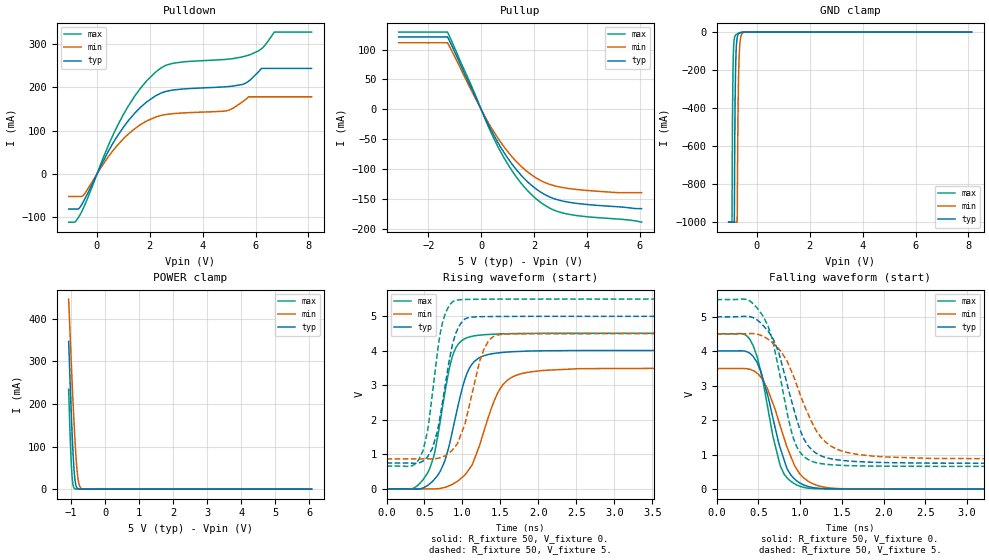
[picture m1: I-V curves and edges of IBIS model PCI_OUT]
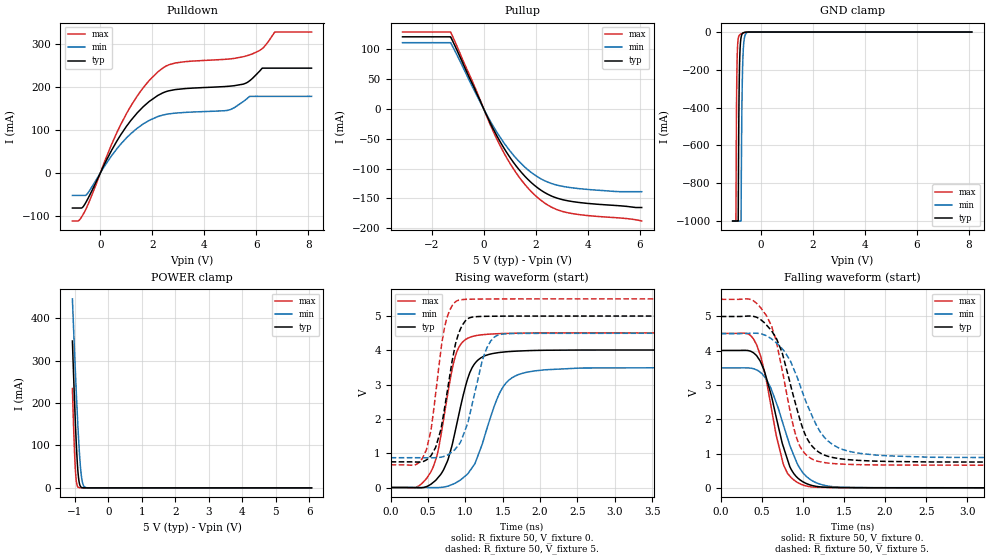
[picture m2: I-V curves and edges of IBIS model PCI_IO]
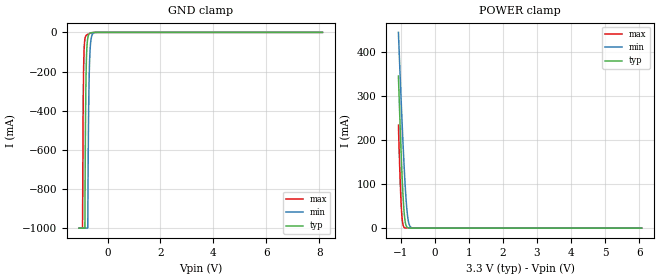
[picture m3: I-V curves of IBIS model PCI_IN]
|   IBIS Model for tsi381
[IBIS Ver]   3.2
[Disclaimer] THIS IBIS MODEL HAS BEEN CREATED BY THE SIGNAL
   INTEGRITY SOFTWARE SPICE-TO-IBIS PROCESS.
   THESE IBIS MODELS ARE PROVIDED "AS IS" WITH NO
   WARRANTY WHATSOEVER AND SIGNAL INTEGRITY SOFTWARE
   SPECIFICALLY DISCLAIMS ANY IMPLIED WARRANTIES OF
   MERCHANTABILITY, FITNESS FOR A PARTICULAR PURPOSE,
   OR AGAINST INFRINGEMENT.
[File Name]   tsi381_pbga_5vpci.ibs
[File Rev]   1.1
[Date]   07/27/2009
[Notes]
   Revision History
   Rev 1.0
   - 2/27/09 Inital Release. IBIS model generated from
   SPICE model extraction. AEP
   Rev 1.1
   - updated it IDT formating. IGT
[Component] tsi381
[Manufacturer] IDT
|   typ   min   max
[Package]
R_pkg   354m   244m   481m
L_pkg   4.50nH   2.81nH   7.01nH
C_pkg   0.86pF   0.64pF   1.33pF
[Pin]  signal_name   model_name   R_pin   L_pin   C_pin
C9   GPIO[0]   NC   299.8m   3.7nh   0.83pf
A10   GPIO[1]   NC   274.4m   3.5nh   0.76pf
B10   GPIO[2]   NC   247.9m   3.3nh   0.64pf
A11   GPIO[3]   NC   287.0m   3.6nh   0.79pf
M2   JTAG_TCK   JTAG_IN   366.2m   4.4nh   0.83pf
L3   JTAG_TDI   JTAG_IN   382.4m   4.9nh   0.94pf
L1   JTAG_TDO   JTAG_OUT   371.7m   4.5nh   0.76pf
M12   JTAG_TMS   JTAG_IN   393.2m   4.5nh   0.85pf
L10   JTAG_TRSTn   JTAG_IN   410.4m   5.3nh   0.96pf
D3   PCI_AD[0]   PCI_IO   398.2m   5.4nh   0.99pf
C1   PCI_AD[1]   PCI_IO   344.1m   4.1nh   0.77pf
F4   PCI_AD[10]   PCI_IO   402.7m   5.8nh   1.06pf
G1   PCI_AD[11]   PCI_IO   310.8m   3.7nh   0.64pf
G2   PCI_AD[12]   PCI_IO   330.2m   4.0nh   0.77pf
G3   PCI_AD[13]   PCI_IO   375.2m   4.9nh   0.90pf
H1   PCI_AD[14]   PCI_IO   311.3m   3.8nh   0.65pf
H2   PCI_AD[15]   PCI_IO   355.7m   4.5nh   0.82pf
J5   PCI_AD[16]   PCI_IO   481.4m   6.8nh   1.29pf
L6   PCI_AD[17]   PCI_IO   343.6m   4.4nh   0.79pf
M6   PCI_AD[18]   PCI_IO   304.3m   3.8nh   0.66pf
K6   PCI_AD[19]   PCI_IO   371.5m   5.1nh   0.92pf
D1   PCI_AD[2]   PCI_IO   330.9m   3.9nh   0.72pf
J6   PCI_AD[20]   PCI_IO   386.3m   5.7nh   1.04pf
M7   PCI_AD[21]   PCI_IO   301.3m   3.7nh   0.65pf
L7   PCI_AD[22]   PCI_IO   326.6m   4.1nh   0.77pf
K7   PCI_AD[23]   PCI_IO   373.6m   4.9nh   0.92pf
L8   PCI_AD[24]   PCI_IO   357.1m   4.4nh   0.81pf
K8   PCI_AD[25]   PCI_IO   437.6m   5.8nh   1.12pf
M9   PCI_AD[26]   PCI_IO   323.3m   3.9nh   0.69pf
L9   PCI_AD[27]   PCI_IO   357.9m   4.5nh   0.84pf
K12   PCI_AD[28]   PCI_IO   346.8m   4.1nh   0.79pf
J11   PCI_AD[29]   PCI_IO   377.8m   4.7nh   0.93pf
D2   PCI_AD[3]   PCI_IO   353.3m   4.5nh   0.85pf
J12   PCI_AD[30]   PCI_IO   324.4m   4.0nh   0.74pf
J10   PCI_AD[31]   PCI_IO   436.5m   5.9nh   1.16pf
E1   PCI_AD[4]   PCI_IO   309.0m   3.7nh   0.67pf
E2   PCI_AD[5]   PCI_IO   352.5m   4.6nh   0.82pf
E3   PCI_AD[6]   PCI_IO   368.0m   5.0nh   0.94pf
E4   PCI_AD[7]   PCI_IO   480.4m   7.0nh   1.32pf
F2   PCI_AD[8]   PCI_IO   343.3m   4.2nh   0.79pf
F3   PCI_AD[9]   PCI_IO   363.1m   4.8nh   0.91pf
F1   PCI_CBEn[0]   PCI_IO   303.6m   3.7nh   0.65pf
H3   PCI_CBEn[1]   PCI_IO   392.2m   5.0nh   0.94pf
K5   PCI_CBEn[2]   PCI_IO   406.7m   5.4nh   1.06pf
M8   PCI_CBEn[3]   PCI_IO   309.0m   3.8nh   0.66pf
D12   PCI_CLK   PCI_IN   328.4m   3.9nh   0.67pf
H10   PCI_CLKO[0]   PCI_OUT   407.4m   5.6nh   1.09pf
C2   PCI_CLKO[1]   PCI_OUT   408.8m   5.2nh   0.95pf
K4   PCI_DEVSELn   PCI_IO   467.5m   6.4nh   1.28pf
M5   PCI_FRAMEn   PCI_IO   317.2m   3.8nh   0.68pf
G10   PCI_GNTn[0]   PCI_IO   377.6m   4.9nh   1.01pf
G9   PCI_GNTn[1]   PCI_OUT   404.4m   5.5nh   1.09pf
F11   PCI_GNTn[2]   PCI_OUT   346.6m   4.4nh   0.82pf
E11   PCI_GNTn[3]   PCI_OUT   340.9m   4.1nh   0.79pf
E12   PCI_INTAn   PCI_IN   321.7m   4.0nh   0.66pf
E9   PCI_INTBn   PCI_IN   395.4m   5.5nh   1.06pf
D11   PCI_INTCn   PCI_IN   380.1m   4.7nh   0.82pf
E10   PCI_INTDn   PCI_IN   390.8m   5.0nh   0.93pf
L5   PCI_IRDYn   PCI_IO   351.2m   4.5nh   0.87pf
M3   PCI_LOCKn   PCI_OUT   333.8m   4.2nh   0.69pf
D10   PCI_M66EN   PCI_IN   420.4m   5.6nh   0.97pf
J1   PCI_PAR   PCI_IO   328.0m   4.0nh   0.66pf
J3   PCI_PERRn   PCI_IO   436.6m   5.7nh   1.06pf
H12   PCI_PMEn   PCI_IN   326.8m   3.9nh   0.74pf
G11   PCI_REQn[0]   PCI_IO   348.8m   4.3nh   0.85pf
H9   PCI_REQn[1]   PCI_IN   420.8m   6.1nh   1.09pf
G12   PCI_REQn[2]   PCI_IN   305.3m   3.7nh   0.68pf
H11   PCI_REQn[3]   PCI_IN   335.4m   4.3nh   0.81pf
F10   PCI_RSTn   PCI_OUT   366.0m   4.9nh   0.90pf
J2   PCI_SERRn   PCI_IO   376.6m   4.8nh   0.83pf
L4   PCI_STOPn   PCI_IO   385.4m   4.9nh   0.95pf
M4   PCI_TRDYn   PCI_IO   326.3m   3.9nh   0.74pf
B12   PCIE_PERSTn   NC   347.3m   4.3nh   0.66pf
B6   PCIE_REFCLK_n   NC   339.4m   4.2nh   1.02pf
A6   PCIE_REFCLK_p   NC   341.4m   4.1nh   1.01pf
B7   PCIE_RXD_n   NC   253.1m   3.1nh   0.75pf
A8   PCIE_RXD_p   NC   266.3m   3.4nh   0.79pf
A4   PCIE_TXD_n   NC   249.7m   3.3nh   0.69pf
B5   PCIE_TXD_p   NC   244.8m   3.0nh   0.69pf
K11   PWRUP_EN_ARB   GEN33_IN   407.8m   5.1nh   1.04pf
M1   PWRUP_PLL_BYPASS   GEN33_IN   410.2m   4.8nh   0.93pf
B2   SR_CLK   NC   418.6m   5.1nh   0.96pf
C4   SR_CSn   NC   412.7m   5.5nh   1.33pf
A2   SR_DIN   NC   308.5m   3.8nh   0.87pf
A1   SR_DOUT   NC   366.1m   4.5nh   0.78pf
C8   TEST_BCE   NC   313.4m   4.3nh   0.96pf
B1   TEST_BIDR_CTL   NC   371.0m   4.4nh   0.80pf
A3   TEST_ON   NC   332.2m   4.3nh   0.93pf
M11   TEST_SPARE[0]   NC   371.4m   4.4nh   0.79pf
D8   TEST_SPARE[1]   NC   252.7m   2.8nh   0.70pf
K1   TEST_SPARE[2]   NC   349.1m   4.3nh   0.71pf
C10   VDD   POWER
D4   VDD   POWER
F6   VDD   POWER
F8   VDD   POWER
G6   VDD   POWER
G7   VDD   POWER
J9   VDD   POWER
K3   VDD   POWER
B3   VDD_PCI   POWER
B11   VDD_PCI   POWER
F9   VDD_PCI   POWER
G4   VDD_PCI   POWER
H5   VDD_PCI   POWER
H8   VDD_PCI   POWER
J7   VDD_PCI   POWER
L2   VDD_PCI   POWER
M10   VDD_PCI   POWER
A5   VDD_PCIE   POWER
A7   VDD_PCIE   POWER
D5   VDD_PCIE   POWER
E5   VDDA_PCIE   POWER
E7   VDDA_PLL   POWER
F5   VIO_PCI   POWER
G8   VIO_PCI   POWER
H6   VIO_PCI   POWER
B8   VSS   GND
B4   VSS   GND
C6   VSS   GND
C5   VSS   GND
D9   VSS   GND
D7   VSS   GND
D6   VSS   GND
E6   VSS   GND
F7   VSS   GND
G5   VSS   GND
H7   VSS   GND
H4   VSS   GND
A12   VSS_IO   GND
C11   VSS_IO   GND
C3   VSS_IO   GND
F12   VSS_IO   GND
J8   VSS_IO   GND
J4   VSS_IO   GND
K10   VSS_IO   GND
K2   VSS_IO   GND
C7   VSSA_PLL   GND
| Models and submodels in the file (6): PCI_OUT (Output), PCI_IO (I/O), PCI_IN (Input), JTAG_IN (Input), JTAG_OUT (Output), GEN33_IN (Input)
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[Model]   PCI_OUT
Model_type  Output
C_comp 4.536p 4.202p 4.874p
Polarity   Non-Inverting
Enable   Active-High
Vmeas =   1.32V
Cref =   10pF
Rref =   50
Vref=   0.0V
[Temperature Range]   27.0   125.0   -40.0
[Voltage Range] 5. 4.5 5.5
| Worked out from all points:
|   slope of the pulldown table from 0 to 0.75 V, typ, clamps not added: 8.81 ohm
|   slope of the pullup table from 0 to 0.75 V, typ, clamps not added: 11.8 ohm
|   GND clamp passes 1 mA (typ) near -0.58 V on its own axis
|   POWER clamp passes 1 mA (typ) near -0.80 V on its own axis
|   rising waveform, R_fixture 50, V_fixture 0.: 20-80 % time 271ps typ, 341ps min, 223ps max; typ from 0 V to 4.01 V
|   rising waveform, R_fixture 50, V_fixture 5.: 20-80 % time 204ps typ, 254ps min, 174ps max; typ from 0.748 V to 5 V
|   falling waveform, R_fixture 50, V_fixture 0.: 20-80 % time 260ps typ, 305ps min, 229ps max; typ from 4.01 V to 0 V
|   falling waveform, R_fixture 50, V_fixture 5.: 20-80 % time 307ps typ, 393ps min, 259ps max; typ from 5 V to 0.748 V
[Pulldown]
-1.072V   -80.93mA   -51.78mA   -111mA
-830.1mV  -80.93mA   -51.78mA   -110.2mA
-625.6mV  -75.05mA   -51.78mA   -92.1mA
425mV     51.67mA    39.35mA    65.16mA
1.011V    108.6mA    81.72mA    138.1mA
2.21V     179.7mA    130.8mA    234.1mA
2.879V    193.3mA    138.9mA    254.9mA
4.887V    200.8mA    145.2mA    263.9mA
5.761V    214.7mA    177.7mA    274.1mA
6.226V    243mA      177.7mA    288.2mA
6.71V     243mA      177.7mA    326.7mA
8.123V    243mA      177.7mA    326.7mA
[Pullup]
-3.123V   121mA      111.2mA    129.1mA
-1.273V   121mA      111.2mA    129.1mA
-408.1mV  39.21mA    34.71mA    43.33mA
103.2mV   -9.96mA    -8.61mA    -11.21mA
754mV     -64.09mA   -55.48mA   -71.94mA
1.433V    -105.7mA   -91.4mA    -118.6mA
1.786V    -121.9mA   -105.2mA   -136.8mA
2.186V    -135.9mA   -116.9mA   -152.8mA
2.725V    -148.2mA   -126.7mA   -167.3mA
3.264V    -154.4mA   -131.5mA   -174.5mA
4.984V    -161.7mA   -138.3mA   -182.2mA
6.072V    -165.4mA   -138.8mA   -188mA
[GND Clamp]
-1.072V   -1A        -1A        -1A
-946.2mV  -1A        -1A        -1A
-927.6mV  -1A        -1A        -477.7mA
-913.6mV  -1A        -1A        -259.6mA
-857.8mV  -1A        -1A        -35.04mA
-829.9mV  -387.1mA   -1A        -20.17mA
-792.7mV  -109.1mA   -1A        -13.52mA
-750.8mV  -31.16mA   -1A        -10.02mA
-718.2mV  -13.49mA   -425.6mA   -7.927mA
-681mV    -5.936mA   -150.7mA   -5.835mA
-541.4mV  -487.9uA   -4.567mA   -875.4uA
8.123V    0A         0A         0A
[Power Clamp]
-1.072V   346.3mA    445.7mA    234.2mA
-1.025V   239mA      352.7mA    117.5mA
-985.9mV  158.9mA    279.6mA    47.19mA
-953.7mV  100.9mA    221.8mA    15.32mA
-930mV    65.56mA    181.6mA    5.554mA
-906.4mV  38.32mA    144mA      1.868mA
-865.6mV  11.54mA    86.96mA    261.8uA
-839.8mV  4.741mA    57.78mA    114.1uA
-809.7mV  1.564mA    32.24mA    114.1uA
-764.6mV  288.3uA    10.74mA    114.1uA
-708.7mV  34.28uA    2.193mA    114.1uA
6.072V    0A         0A         0A
[Ramp]
dV/dt_r 2.406/269.779p 2.1/340.819p 2.705/222.777p
dV/dt_f 2.551/306.834p 2.179/393.351p 2.904/258.7p
[Rising Waveform]
R_fixture = 50
V_fixture = 0.
0s        0V         0V         0V
340ps     -4.676mV   86.06uV    4.549mV
540ps     94.69mV    -2.304mV   456.9mV
640ps     301mV      -2.262mV   1.113V
770ps     822.3mV    41.22mV    2.797V
860ps     1.592V     120.4mV    3.781V
1.06ns    3.349V     481.1mV    4.379V
1.46ns    3.937V     2.758V     4.487V
1.71ns    3.979V     3.291V     4.5V
4.91ns    4.01V      3.5V       4.508V
[Rising Waveform]
R_fixture = 50
V_fixture = 5.
V_fixture_min = 4.5
V_fixture_max = 5.5
0s        748.2mV    868.5mV    660.9mV
340ps     743.4mV    868.5mV    668.5mV
480ps     805.4mV    867.5mV    1.103V
610ps     1.216V     870.6mV    2.858V
720ps     2.281V     911.3mV    4.647V
890ps     4.347V     1.186V     5.445V
1.03ns    4.918V     1.86V      5.488V
1.28ns    4.991V     4.027V     5.496V
1.43ns    4.995V     4.436V     5.498V
4.91ns    5V         4.5V       5.5V
[Falling Waveform]
R_fixture = 50
V_fixture = 0.
0s        4.01V      3.5V       4.508V
400ps     3.94V      3.477V     4.342V
530ps     3.418V     3.25V      3.403V
670ps     2.118V     2.522V     1.6V
760ps     1.216V     1.855V     703.3mV
860ps     527.8mV    1.121V     291.2mV
990ps     192.2mV    470.5mV    92.32mV
1.17ns    40.8mV     141mV      16.71mV
1.44ns    9.292mV    19.45mV    6.614mV
4.91ns    8.688uV    23.08uV    4.321uV
[Falling Waveform]
R_fixture = 50
V_fixture = 5.
V_fixture_min = 4.5
V_fixture_max = 5.5
0s        5V         4.5V       5.5V
370ps     5.012V     4.511V     5.491V
560ps     4.742V     4.432V     5.006V
670ps     4.387V     4.245V     4.331V
740ps     3.99V      4.079V     3.529V
920ps     2.368V     3.287V     1.483V
1.14ns    1.146V     1.95V      809.5mV
1.37ns    882.2mV    1.249V     708.4mV
1.71ns    797.4mV    1.002V     675.1mV
4.91ns    748.3mV    869.1mV    660.9mV
[Model]   PCI_IO
Model_type  I/O
C_comp 4.536p 4.202p 4.874p
Polarity   Non-Inverting
Enable   Active-High
Vinl =   0.80V
Vinh =   2.00V
Vmeas =   1.32V
Cref =   10pF
Rref =   150
Vref=   0.0V
[Temperature Range]   27.0   125.0   -40.0
[Voltage Range] 5. 4.5 5.5
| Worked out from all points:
|   slope of the pulldown table from 0 to 0.75 V, typ, clamps not added: 8.81 ohm
|   slope of the pullup table from 0 to 0.75 V, typ, clamps not added: 11.8 ohm
|   GND clamp passes 1 mA (typ) near -0.58 V on its own axis
|   POWER clamp passes 1 mA (typ) near -0.80 V on its own axis
|   rising waveform, R_fixture 50, V_fixture 0.: 20-80 % time 271ps typ, 341ps min, 223ps max; typ from 0 V to 4.01 V
|   rising waveform, R_fixture 50, V_fixture 5.: 20-80 % time 204ps typ, 254ps min, 174ps max; typ from 0.748 V to 5 V
|   falling waveform, R_fixture 50, V_fixture 0.: 20-80 % time 260ps typ, 305ps min, 229ps max; typ from 4.01 V to 0 V
|   falling waveform, R_fixture 50, V_fixture 5.: 20-80 % time 307ps typ, 393ps min, 259ps max; typ from 5 V to 0.748 V
[Pulldown]
-1.072V   -80.93mA   -51.78mA   -111mA
-830.1mV  -80.93mA   -51.78mA   -110.2mA
-625.6mV  -75.05mA   -51.78mA   -92.1mA
425mV     51.67mA    39.35mA    65.16mA
1.011V    108.6mA    81.72mA    138.1mA
2.21V     179.7mA    130.8mA    234.1mA
2.879V    193.3mA    138.9mA    254.9mA
4.887V    200.8mA    145.2mA    263.9mA
5.761V    214.7mA    177.7mA    274.1mA
6.226V    243mA      177.7mA    288.2mA
6.71V     243mA      177.7mA    326.7mA
8.123V    243mA      177.7mA    326.7mA
[Pullup]
-3.123V   121mA      111.2mA    129.1mA
-1.273V   121mA      111.2mA    129.1mA
-408.1mV  39.21mA    34.71mA    43.33mA
103.2mV   -9.96mA    -8.61mA    -11.21mA
754mV     -64.09mA   -55.48mA   -71.94mA
1.433V    -105.7mA   -91.4mA    -118.6mA
1.786V    -121.9mA   -105.2mA   -136.8mA
2.186V    -135.9mA   -116.9mA   -152.8mA
2.725V    -148.2mA   -126.7mA   -167.3mA
3.264V    -154.4mA   -131.5mA   -174.5mA
4.984V    -161.7mA   -138.3mA   -182.2mA
6.072V    -165.4mA   -138.8mA   -188mA
[GND Clamp]
-1.072V   -1A        -1A        -1A
-946.2mV  -1A        -1A        -1A
-927.6mV  -1A        -1A        -477.7mA
-913.6mV  -1A        -1A        -259.6mA
-857.8mV  -1A        -1A        -35.04mA
-829.9mV  -387.1mA   -1A        -20.17mA
-792.7mV  -109.1mA   -1A        -13.52mA
-750.8mV  -31.16mA   -1A        -10.02mA
-718.2mV  -13.49mA   -425.6mA   -7.927mA
-681mV    -5.936mA   -150.7mA   -5.835mA
-541.4mV  -487.9uA   -4.567mA   -875.4uA
8.123V    0A         0A         0A
[Power Clamp]
-1.072V   346.3mA    445.7mA    234.2mA
-1.025V   239mA      352.7mA    117.5mA
-985.9mV  158.9mA    279.6mA    47.19mA
-953.7mV  100.9mA    221.8mA    15.32mA
-930mV    65.56mA    181.6mA    5.554mA
-906.4mV  38.32mA    144mA      1.868mA
-865.6mV  11.54mA    86.96mA    261.8uA
-839.8mV  4.741mA    57.78mA    114.1uA
-809.7mV  1.564mA    32.24mA    114.1uA
-764.6mV  288.3uA    10.74mA    114.1uA
-708.7mV  34.28uA    2.193mA    114.1uA
6.072V    0A         0A         0A
[Ramp]
dV/dt_r 2.406/269.779p 2.1/340.819p 2.705/222.777p
dV/dt_f 2.551/306.834p 2.179/393.351p 2.904/258.7p
[Rising Waveform]
R_fixture = 50
V_fixture = 0.
0s        0V         0V         0V
340ps     -4.676mV   86.06uV    4.549mV
540ps     94.69mV    -2.304mV   456.9mV
640ps     301mV      -2.262mV   1.113V
770ps     822.3mV    41.22mV    2.797V
860ps     1.592V     120.4mV    3.781V
1.06ns    3.349V     481.1mV    4.379V
1.46ns    3.937V     2.758V     4.487V
1.71ns    3.979V     3.291V     4.5V
4.91ns    4.01V      3.5V       4.508V
[Rising Waveform]
R_fixture = 50
V_fixture = 5.
V_fixture_min = 4.5
V_fixture_max = 5.5
0s        748.2mV    868.5mV    660.9mV
340ps     743.4mV    868.5mV    668.5mV
480ps     805.4mV    867.5mV    1.103V
610ps     1.216V     870.6mV    2.858V
720ps     2.281V     911.3mV    4.647V
890ps     4.347V     1.186V     5.445V
1.03ns    4.918V     1.86V      5.488V
1.28ns    4.991V     4.027V     5.496V
1.43ns    4.995V     4.436V     5.498V
4.91ns    5V         4.5V       5.5V
[Falling Waveform]
R_fixture = 50
V_fixture = 0.
0s        4.01V      3.5V       4.508V
400ps     3.94V      3.477V     4.342V
530ps     3.418V     3.25V      3.403V
670ps     2.118V     2.522V     1.6V
760ps     1.216V     1.855V     703.3mV
860ps     527.8mV    1.121V     291.2mV
990ps     192.2mV    470.5mV    92.32mV
1.17ns    40.8mV     141mV      16.71mV
1.44ns    9.292mV    19.45mV    6.614mV
4.91ns    8.688uV    23.08uV    4.321uV
[Falling Waveform]
R_fixture = 50
V_fixture = 5.
V_fixture_min = 4.5
V_fixture_max = 5.5
0s        5V         4.5V       5.5V
370ps     5.012V     4.511V     5.491V
560ps     4.742V     4.432V     5.006V
670ps     4.387V     4.245V     4.331V
740ps     3.99V      4.079V     3.529V
920ps     2.368V     3.287V     1.483V
1.14ns    1.146V     1.95V      809.5mV
1.37ns    882.2mV    1.249V     708.4mV
1.71ns    797.4mV    1.002V     675.1mV
4.91ns    748.3mV    869.1mV    660.9mV
|   MODEL PCI_IN
[Model]   PCI_IN
Model_type  Input
C_comp 4.536p 4.202p 4.874p
Polarity   Non-Inverting
Enable   Active-High
Vinl =   0.80V
Vinh =   2.00V
[Temperature Range]   27.0   125.0   -40.0
[POWER Clamp Reference]   3.30V   3.00V   3.60V
[GND Clamp Reference]   0.00V   0.00V   0.00V
[Voltage Range] 3.3 3. 3.6
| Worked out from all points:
|   GND clamp passes 1 mA (typ) near -0.58 V on its own axis
|   POWER clamp passes 1 mA (typ) near -0.80 V on its own axis
[GND Clamp]
-1.072V   -1A        -1A        -1A
-946.2mV  -1A        -1A        -1A
-927.6mV  -1A        -1A        -477.7mA
-913.6mV  -1A        -1A        -259.6mA
-857.8mV  -1A        -1A        -35.04mA
-829.9mV  -387.1mA   -1A        -20.17mA
-792.7mV  -109.1mA   -1A        -13.52mA
-750.8mV  -31.16mA   -1A        -10.02mA
-718.2mV  -13.49mA   -425.6mA   -7.927mA
-681mV    -5.936mA   -150.7mA   -5.835mA
-541.4mV  -487.9uA   -4.567mA   -875.4uA
8.123V    0A         0A         0A
[Power Clamp]
-1.072V   346.3mA    445.7mA    234.2mA
-1.025V   239mA      352.7mA    117.5mA
-985.9mV  158.9mA    279.6mA    47.19mA
-953.7mV  100.9mA    221.8mA    15.32mA
-930mV    65.56mA    181.6mA    5.554mA
-906.4mV  38.32mA    144mA      1.868mA
-865.6mV  11.54mA    86.96mA    261.8uA
-839.8mV  4.741mA    57.78mA    114.1uA
-809.7mV  1.564mA    32.24mA    114.1uA
-764.6mV  288.3uA    10.74mA    114.1uA
-708.7mV  34.28uA    2.193mA    114.1uA
6.072V    0A         0A         0A
